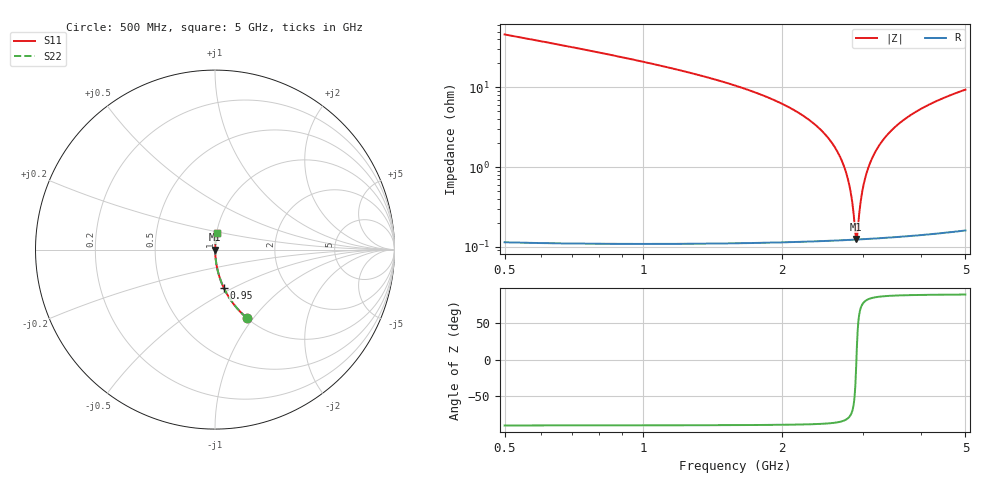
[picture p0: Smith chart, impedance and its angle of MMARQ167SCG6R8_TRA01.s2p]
! MMARQ167SCG6R8_TRA01  S-PARAMETER MODEL  ( General Type )
! Model Generated by TAIYO YUDEN Corporation (http://www.ty-top.com)
! Version 1.0
! TAIYO YUDEN Control No. 150305
! Copyright(c) 2015 TAIYO YUDEN CO.,LTD. All Rights Reserved.
! Product Description (link to TY-COMPAS)
! https://ds.yuden.co.jp/TYCOMPAS/or/detail?pn=MMARQ167SCG6R8CTRA01&u=M
! Products Name : Multilayer Ceramic Capacitors
! Characteristics :
!  Capacitance : 6.8 pF , Rated Voltage : 250V , TCC : CG / C0G
!  Case Size : 1.6 x 0.8 / 0.063 x 0.031 [mm/inch] , Thickness : 0.7 / 0.028 [mm/inch]
!  (Conditions: Temperature = 25 degC , DC Bias Current/Voltage = 0A / 0V)
! External Node Assignments :
!  1  o---| |---o  2
! GND o---------o GND
! Frequency Range : 500MHz  -  5GHz  [ 401 STEP ]
# MHz S RI R 50
! Freq[MHz].  S11 Real  S11 Imag  S21 Real  S21 Imag  S12 Real  S12 Imag  S22 Real  S22 Imag
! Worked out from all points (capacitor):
!   401 points, 500 MHz to 5 GHz, reference 50 ohm
!   read as one part in series: C = 6.71 pF near 522.5 MHz
!   lowest |Z| = 125 mohm at 2.896 GHz (marker M1)
!   series resonance near 2.9 GHz, so ESL is about 450 pH
!   S11 on the Smith chart (normalised r, x): 500 MHz: 1.00, -0.92; 950 MHz: 1.00, -0.45; 5 GHz: 1.00, +0.19
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500  0.1756 -0.3792  0.8244 0.3792  0.8244 0.3792  0.1756 -0.3792
950  0.0483 -0.212  0.9517 0.212  0.9517 0.212  0.0483 -0.212
1253.75  0.0242 -0.15  0.9758 0.15  0.9758 0.15  0.0242 -0.15
2007.5  0.0049 -0.0612  0.9951 0.0612  0.9951 0.0612  0.0049 -0.0612
2277.5  0.00275 -0.0398  0.9973 0.0398  0.9973 0.0398  0.00275 -0.0398
2491.25  0.0018 -0.0249  0.9982 0.0249  0.9982 0.0249  0.0018 -0.0249
2637.5  0.00144 -0.0155  0.9986 0.0155  0.9986 0.0155  0.00144 -0.0155
2750  0.00129 -0.00869  0.9987 0.00869  0.9987 0.00869  0.00129 -0.00869
2817.5  0.00124 -0.00473  0.9988 0.00473  0.9988 0.00473  0.00124 -0.00473
2840  0.00123 -0.00343  0.9988 0.00343  0.9988 0.00343  0.00123 -0.00343
2885  0.00123 -0.000869  0.9988 0.000869  0.9988 0.000869  0.00123 -0.000869
2896.25  0.00123 -0.000233  0.9988 0.000233  0.9988 0.000233  0.00123 -0.000233
2918.75  0.00123 0.00103  0.9988 -0.00103  0.9988 -0.00103  0.00123 0.00103
2963.75  0.00125 0.00353  0.9987 -0.00353  0.9987 -0.00353  0.00125 0.00353
2997.5  0.00127 0.00538  0.9987 -0.00538  0.9987 -0.00538  0.00127 0.00538
3042.5  0.00131 0.00781  0.9987 -0.00781  0.9987 -0.00781  0.00131 0.00781
3098.75  0.00137 0.0108  0.9986 -0.0108  0.9986 -0.0108  0.00137 0.0108
3267.5  0.00166 0.0195  0.9983 -0.0195  0.9983 -0.0195  0.00166 0.0195
3503.75  0.00228 0.031  0.9977 -0.031  0.9977 -0.031  0.00228 0.031
3830  0.00348 0.0459  0.9965 -0.0459  0.9965 -0.0459  0.00348 0.0459
4257.5  0.00555 0.0639  0.9944 -0.0639  0.9944 -0.0639  0.00555 0.0639
5000  0.0102 0.0925  0.9898 -0.0925  0.9898 -0.0925  0.0102 0.0925
